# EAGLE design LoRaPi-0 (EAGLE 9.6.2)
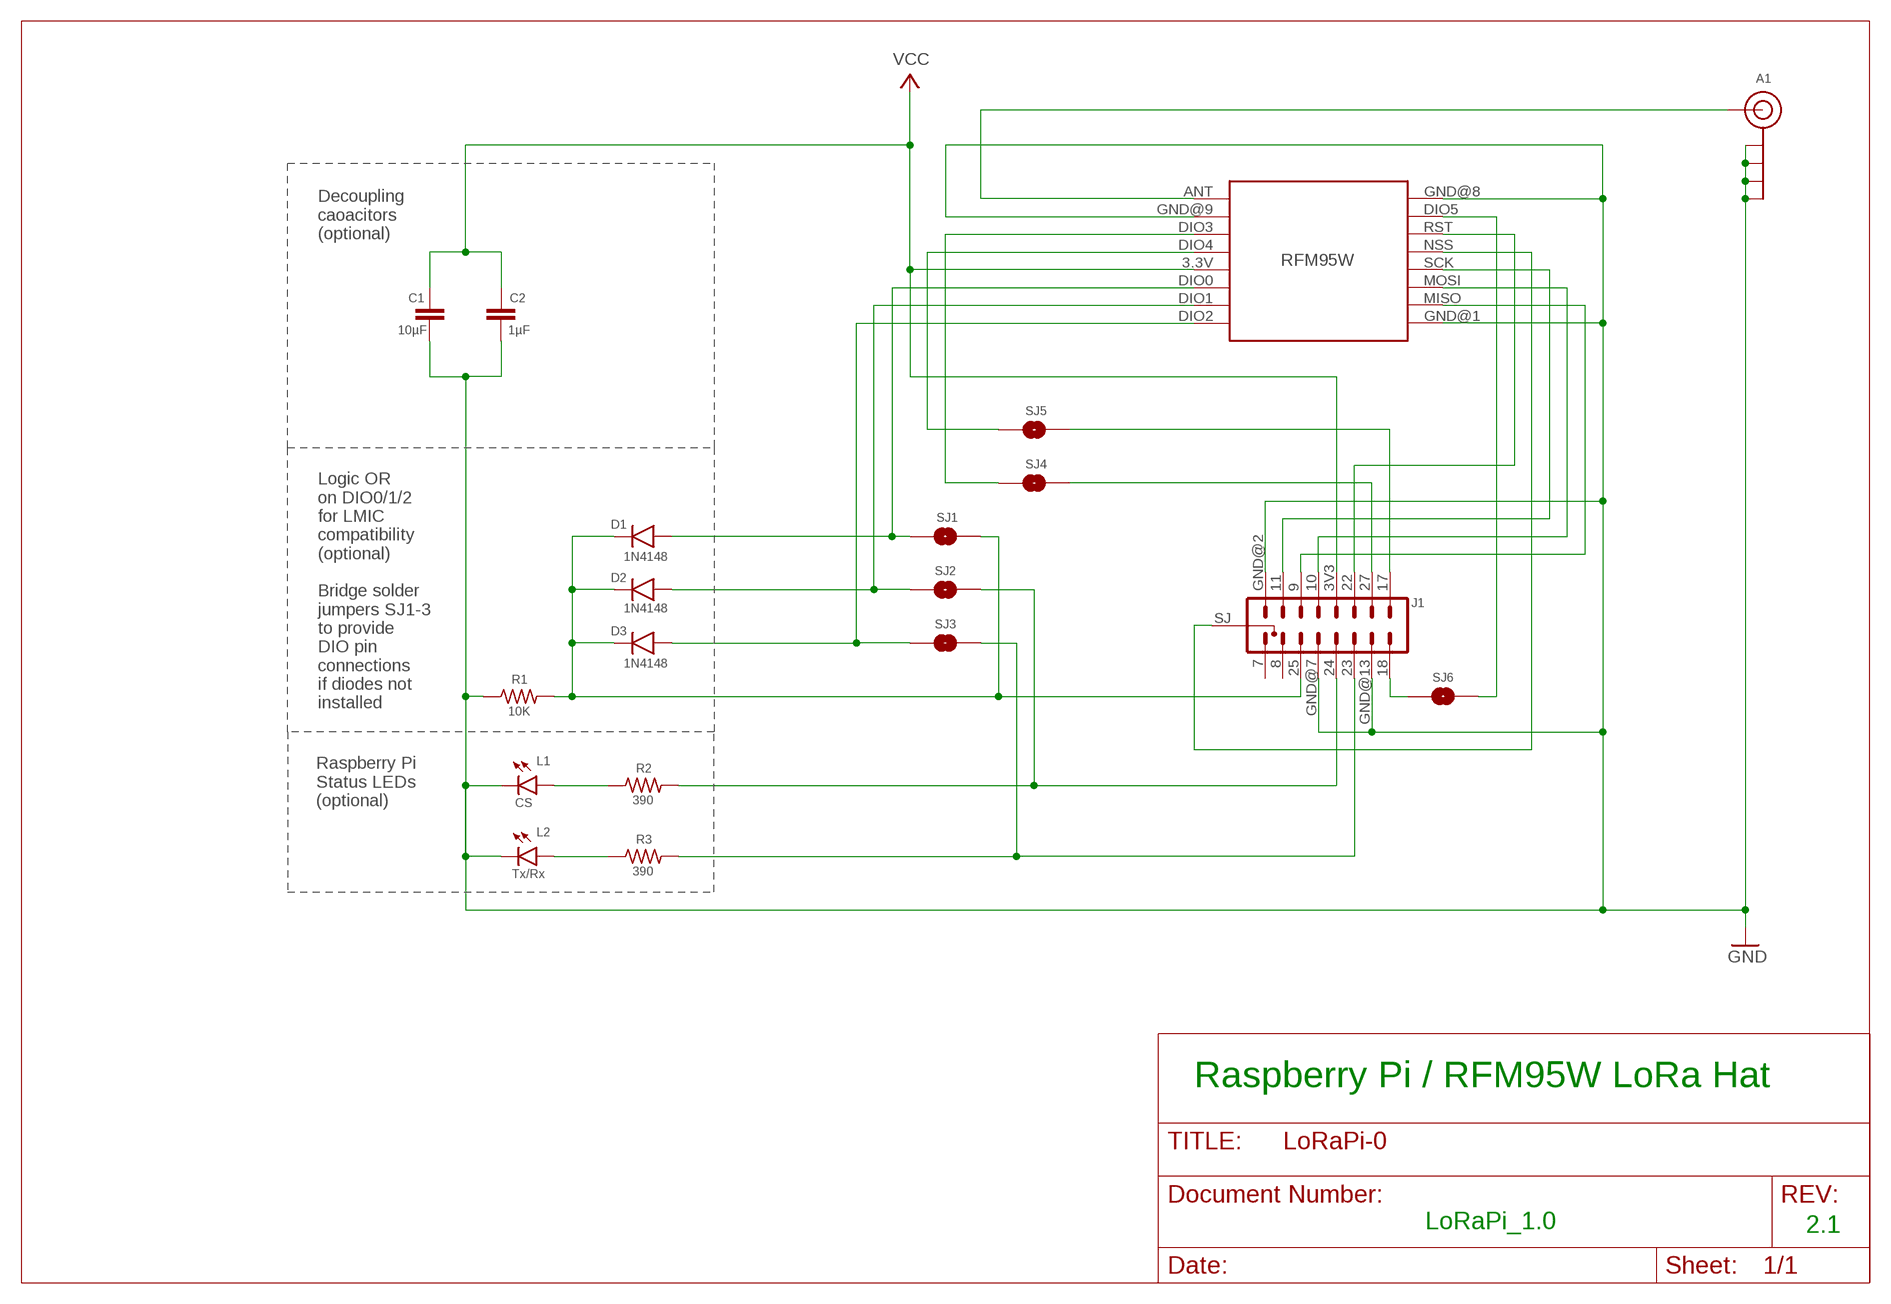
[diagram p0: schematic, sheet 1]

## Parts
A1  U.FL-SMA-EDGE-COMBO  [U.FL-SMA-EDGE-COMBO]
C1  10µF  CAPACITOR  [C0805]
C2  1µF  CAPACITOR  [C0805]
D1  1N4148  1N4148SMD  [SOD-123]
D2  1N4148  1N4148SMD  [SOD-123]
D3  1N4148  1N4148SMD  [SOD-123]
J1  HEADER-2X8-RFM95W-PI  [CONN_2X8-RFM-PI]
L1  CS  LEDCHIP-LED0805  [CHIP-LED0805]
L2  Tx/Rx  LEDCHIP-LED0805  [CHIP-LED0805]
R1  10K  R-US_R0805  [R0805]
R2  390  R-US_R0805  [R0805]
R3  390  R-US_R0805  [R0805]
RFM95W  RFM95W-LORA  [RFM95W-LORA]
SJ1  SJ  [SJ]
SJ2  SJ  [SJ]
SJ3  SJ  [SJ]
SJ4  SJ  [SJ]
SJ5  SJ  [SJ]
SJ6  SJ  [SJ]

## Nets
GND: A1.GND@1A(GND) A1.GND@1B(GND) A1.GND@2A(GND) A1.GND@2B(GND) C1.2 C2.2 J1.GND@2 J1.GND@7 J1.GND@13 L1.C L2.C R1.1 RFM95W.GND@1(GND.1) RFM95W.GND@8(GND.2) RFM95W.GND@9(GND.3)
N$1: L2.A R3.1
N$2: L1.A R2.1
N$3: J1.18 SJ6.1
N$4: J1.SJ(8-9) RFM95W.NSS
N$5: J1.23 R3.2 SJ3.2
N$6: J1.24 R2.2 SJ2.2
N$7: D1.2 RFM95W.DIO0 SJ1.1
N$8: RFM95W.DIO4 SJ5.1
N$9: RFM95W.DIO3 SJ4.1
N$10: D1.1 D2.1 D3.1 J1.25 R1.2 SJ1.2
N$11: A1.SIG RFM95W.ANT
N$12: D2.2 RFM95W.DIO1 SJ2.1
N$13: J1.22 RFM95W.RST
N$14: D3.2 RFM95W.DIO2 SJ3.1
N$15: J1.11 RFM95W.SCK
N$16: J1.10 RFM95W.MOSI
N$17: J1.9 RFM95W.MISO
N$18: J1.27 SJ4.2
N$19: J1.17 SJ5.2
N$20: RFM95W.DIO5 SJ6.2
VCC: C1.1 C2.1 J1.3V3 RFM95W.3.3V
Unconnected: J1.7 J1.8

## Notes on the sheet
- Decoupling
  caoacitors
  (optional)
- Logic OR
  on DIO0/1/2
  for LMIC
  compatibility
  (optional)
  
  Bridge solder
  jumpers SJ1-3
  to provide
  DIO pin
  connections
  if diodes not
  installed
- Raspberry Pi
  Status LEDs
  (optional)
- Raspberry Pi / RFM95W LoRa Hat
- LoRaPi_1.0 | 2.1

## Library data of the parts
A1 = digitalconcepts:U.FL-SMA-EDGE-COMBO: Combination u.FL & SMA edge mount antenna
C1 C2 = digitalconcepts:CAPACITOR: 0805 Capacitor
D1-D3 = digitalconcepts:1N4148: 1N4148 SOD-123 Signal Diode
J1 = digitalconcepts:HEADER-2X8-RFM95W-PI: PI-RFM95W 2x16 Pin Header for Raspberry Pi RFM95W daughter baord
L1 L2 = led:LED: LED
R1-R3 = digitalconcepts:R-US_: RESISTOR, American symbol; SPICEPREFIX: R
RFM95W = digitalconcepts:RFM95W-LORA: RFM95W LoRa Wireless Transceiver
SJ1-SJ6 = digitalconcepts:SJ: Solder Jumper

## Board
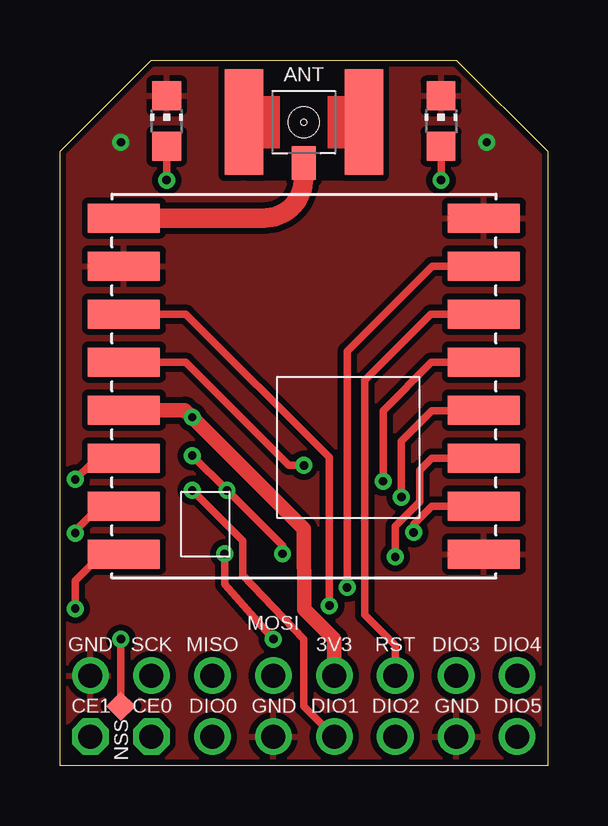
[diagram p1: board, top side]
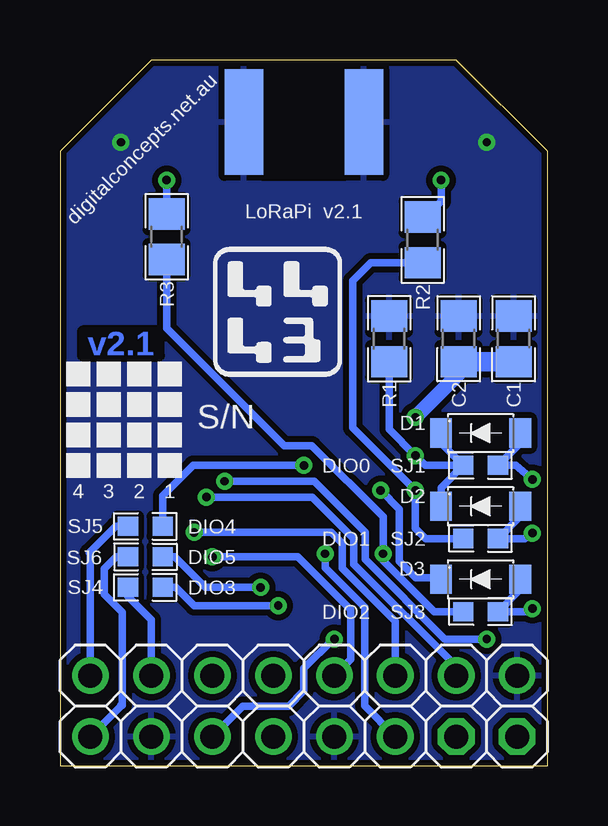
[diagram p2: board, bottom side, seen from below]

Size 20.32 x 29.4 mm. Coordinates in mm from the lower left corner, seen from the top.
Outline: 0,0 0,25.59 3.81,29.4 16.51,29.4 20.32,25.59 20.32,0 0,0
Copper layers (1*16): Top 0.0356mm / dielectric 1.5011mm / Bottom 0.0356mm
Design rules "PCBs_io *": minimum track width 6mil, minimum drill 13mil, track to track 6mil, track to pad 6mil, pad to pad 6mil, via to via 6mil, smd to smd 6mil, copper to edge 6mil, drill to drill 6mil, minimum pad ring 7mil, minimum via ring 7mil, stop-mask expansion 3mil, vias tented up to drill 0mil, thermal gap 10mil

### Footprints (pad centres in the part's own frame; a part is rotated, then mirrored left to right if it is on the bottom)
U.FL-SMA-EDGE-COMBO = smd 1.6 x 4.4: GND@1A -2.5,0; GND@2A 2.5,0 | smd 1.6 x 4.4 bottom: GND@1B -2.5,0; GND@2B 2.5,0 | smd 1 x 1.4: SIG 0,-1.7
C0805 = smd 1.3 x 1.5: 1 -0.95,0; 2 0.95,0
SOD-123 = smd 0.91 x 1.22: 1 1.65,0; 2 -1.65,0
CONN_2X8-RFM-PI = drill 1 pad 1.524: 3V3 7.62,2.54; 9 2.54,2.54; 10 5.08,2.54; 11 0,2.54; 17 15.24,2.54; 18 15.24,0; 22 10.16,2.54; 23 10.16,0; 24 7.62,0; 25 2.54,0; 27 12.7,2.54; GND@2 -2.54,2.54; GND@7 5.08,0; GND@13 12.7,0 | drill 1 pad 1.524 octagon: 7 -2.54,0; 8 0,0 | smd 0.864 x 0.864 rotated 45: SJ -1.27,1.27
CHIP-LED0805 = smd 1.2 x 1.2: A 0,-1.05; C 0,1.05
R0805 = smd 1.3 x 1.5: 1 -0.95,0; 2 0.95,0
RFM95W-LORA = smd 3 x 1.2: 3.3V 7.5,1; ANT 7.5,-7; DIO0 7.5,3; DIO1 7.5,5; DIO2 7.5,7; DIO3 7.5,-3; DIO4 7.5,-1; DIO5 -7.5,-5; GND@1 -7.5,7; GND@8 -7.5,-7; GND@9 7.5,-5; MISO -7.5,5; MOSI -7.5,3; NSS -7.5,-1; RST -7.5,-3; SCK -7.5,1
SJ = smd 0.85 x 0.8: 1 -0.725,0; 2 0.725,0

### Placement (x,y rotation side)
A1  10.16,26.81 0 top
C1  1.42,17.78 90 bottom
C2  3.71,17.78 90 bottom
D1  2.79,13.86 180 bottom
D2  2.79,10.81 180 bottom
D3  2.79,7.76 180 bottom
J1  3.81,1.21 0 top
L1  4.45,26.86 0 top
L2  15.88,26.86 0 top
R1  6.6,17.78 270 bottom
R2  5.21,21.91 270 bottom
R3  15.88,22.03 270 bottom
RFM95W  10.16,15.81 180 top
SJ1  2.79,12.51 180 bottom
SJ2  2.79,9.46 180 bottom
SJ3  2.79,6.41 180 bottom
SJ4  16.76,7.43 180 bottom
SJ5  16.76,9.97 180 bottom
SJ6  16.76,8.7 0 bottom

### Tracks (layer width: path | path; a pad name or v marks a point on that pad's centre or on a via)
GND  (via drill 0.35)
  other vias: 2.54,25.97 17.78,25.97
  pour Top (isolate 0.254): 3.56,30.42 16.64,30.42 21.46,25.59 21.46,-0.83 -1.02,-0.83 -1.02,25.84
  pour Bottom (isolate 0.254): 3.81,29.53 16.51,29.53 20.57,25.46 20.57,-0.06 -0.25,-0.06 -0.25,25.46
N$1  (via drill 0.35)
  Top 0.305: L2.A v15.88,24.4
  Bottom 0.305: v15.88,24.4 R3.1
N$2  (via drill 0.35)
  Top 0.305: L1.A v4.45,24.4
  Bottom 0.305: v4.45,24.4 4.45,23.51 5.08,22.87 R2.1
N$3
  Bottom 0.305: SJ6.1 17.98,8.7 18.47,8.21 18.47,7.13 17.73,6.39 17.73,2.52 17.78,2.52 17.78,2.47 J1.18
N$4  (via drill 0.35)
  Top 0.305: v13.46,11.85 13.46,14.8 15.48,16.81 RFM95W.NSS | v2.54,5.27 J1.SJ
  Bottom 0.305: v13.46,11.85 9.73,11.85 7.59,9.71 7.59,8.6 4.29,5.27 v2.54,5.27
N$5  (via drill 0.35)
  Top 0.305: v6.86,8.83 6.86,7.56 v8.89,5.27
  Bottom 0.305: SJ3.2 4.73,6.41 6.86,8.54 v6.86,8.83 6.86,10.36 9.82,13.33 10.98,13.33 15.88,18.22 R3.2 | v8.89,5.27 8.94,5.27 10.16,4.05 10.16,3.11 10.8,2.48 12.7,2.48 J1.23
N$6  (via drill 0.35)
  Top 0.305: v5.51,11.47 7.62,9.36 7.62,7.94 10.16,5.27 10.16,2.48 J1.24
  Bottom 0.305: SJ2.2 5.08,9.46 5.51,9.9 v5.51,11.47 8.13,14.08 8.13,20.2 7.37,20.96 R2.2
N$7  (via drill 0.35)
  Top 0.305: v0.63,11.93 1.95,13.19 RFM95W.DIO0
  Bottom 0.305: v0.63,11.93 1.32,12.51 SJ1.1 1.14,13.43 D1.2
N$8  (via drill 0.35)
  Top 0.305: RFM95W.DIO4 5.23,16.81 9.53,12.51 v10.16,12.51
  Bottom 0.305: v10.16,12.51 14.78,12.51 16.04,11.25 SJ5.1
N$9  (via drill 0.35)
  Top 0.305: v11.23,6.67 11.23,12.85 5.23,18.81 RFM95W.DIO3
  Bottom 0.305: SJ4.1 15.49,7.43 14.73,6.67 v11.23,6.67
N$10  (via drill 0.35)
  Top 0.305: v5.51,12.92 v6.96,11.47 9.27,9.16 v9.27,8.83
  Bottom 0.152: D3.1 4.51,7.83
  Bottom 0.305: v9.27,8.83 9.27,8.24 7.62,6.59 7.62,2.49 J1.25 | SJ1.2 4.44,11.58 D2.1 | D1.1 4.44,13.43 SJ1.2 | 4.51,7.83 5.49,7.83 6.17,8.51 6.17,10.68 v6.96,11.47 | R1.2 6.6,14.01 v5.51,12.92 5.1,12.51 SJ1.2
N$11
  Top 0.813: A1.SIG 10.16,24.6 10.15,24.47 arc-90 8.49,22.81 RFM95W.ANT
N$12  (via drill 0.35)
  Top 0.305: RFM95W.DIO1 2.03,11.19 0.63,9.79 v0.63,9.69
  Bottom 0.305: v0.63,9.69 0.96,9.46 SJ2.1 1.14,10.39 D2.2
N$13
  Top 0.305: RFM95W.RST 15.45,18.81 12.7,16.07 12.7,6.29 13.97,5.02 J1.22
N$14  (via drill 0.35)
  Top 0.305: RFM95W.DIO2 2.12,9.19 0.63,7.71 v0.63,6.54
  Bottom 0.305: v0.63,6.54 0.86,6.41 SJ3.1 1.14,7.34 D3.2
N$15  (via drill 0.35)
  Top 0.305: v14.22,11.19 14.22,13.53 15.49,14.8 17.26,14.8 RFM95W.SCK
  Bottom 0.305: v14.22,11.19 9.8,11.19 8.08,9.46 8.08,8.39 3.81,4.14 J1.11
N$16  (via drill 0.35)
  Top 0.305: RFM95W.MOSI 15.49,12.81 14.99,12.3 14.99,10.99 13.97,9.97 v13.97,8.7
  Bottom 0.305: v13.97,8.7 10.41,8.7 8.2,6.49 8.2,4.43 J1.10
N$17  (via drill 0.35)
  Top 0.305: RFM95W.MISO 15.49,10.81 14.73,10.05 v14.73,9.72
  Bottom 0.305: v14.73,9.72 9.02,9.72 8.56,9.25 8.56,8.22 6.35,6.01 J1.9
N$18
  Bottom 0.305: SJ4.2 17.49,7.05 16.51,6.07 J1.27
N$19
  Bottom 0.305: SJ5.2 18,9.97 19.09,8.87 19.05,8.83 J1.17
N$20  (via drill 0.35)
  Top 0.305: v11.96,7.43 11.96,17.26 15.51,20.81 RFM95W.DIO5
  Bottom 0.305: SJ6.2 15.53,8.7 14.26,7.43 v11.96,7.43
VCC  (via drill 0.35)
  Top 0.305: 10.16,9.86 10.16,9.84
  Top 0.61: 10.16,9.84 10.19,6.54 10.19,6.52 11.43,5.27 J1.3V3 | RFM95W.3.3V 5.2,14.81 v5.5,14.51 v5.51,14.52 10.16,9.86
  Bottom 0.61: C2.1 3.71,16.32 v5.51,14.52
  Bottom 0.813: C1.1 C2.1

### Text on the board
Bottom: v2.1
tPlace: ANT
bPlace: digitalconcepts.net.au | LoRaPi v2.1 | S/N | 1 | 2 | 3 | 4
tNames: MOSI | GND | SCK | MISO | 3V3 | RST | DIO3 | DIO4 | CE1 | CE0 | DIO0 | GND | DIO1 | DIO2 | GND | DIO5 | NSS
bNames: DIO0 | DIO4 | DIO1 | DIO5 | DIO3 | DIO2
